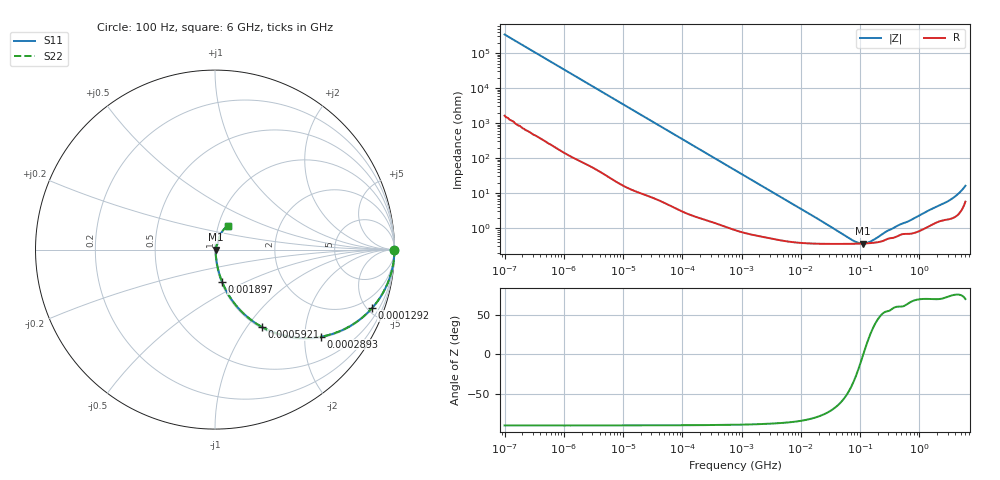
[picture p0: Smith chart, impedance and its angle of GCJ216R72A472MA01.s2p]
!Murata Part Number: GCJ216R72A472MA01
!These Parameters are Measured in Series Mode Connection
!Data Generated on Mar 13, 2026
!  o--ll--o
!Port1  Port2
!  o------o
!Operation Temp=25[degC], DC Bias Voltage=0[V]
!Freq. Start=100[Hz] Stop=6[GHz] 401[Steps]
# Hz S RI R 50
!Freq.(Hz) S11(Real) S11(Imag) S21(Real) S21(Imag) S12(Real) S12(Imag) S22(Real) S22(Imag)
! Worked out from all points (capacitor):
!   401 points, 100 Hz to 6 GHz, reference 50 ohm
!   read as one part in series: C = 4.69 nF near 109 Hz
!   lowest |Z| = 363 mohm at 111.6 MHz (marker M1)
!   series resonance near 113.6 MHz, so ESL is about 420 pH
!   S11 on the Smith chart (normalised r, x): 100 Hz: open; 129.2 kHz: 1.05, -5.37; 289.3 kHz: 1.03, -2.41; 592.1 kHz: 1.02, -1.18; 1.897 MHz: 1.01, -0.37; 6 GHz: 1.11, +0.30
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100  1 -0.000295  1.5e-06 0.000295  1.5e-06 0.000295  1 -0.000295
2008  0.9999 -0.00587  6.11e-05 0.00587  6.11e-05 0.00587  0.9999 -0.00587
12592  0.9985 -0.0366  0.00152 0.0366  0.00152 0.0366  0.9985 -0.0366
40335  0.9857 -0.1151  0.0143 0.1151  0.0143 0.1151  0.9857 -0.1151
78952  0.949 -0.216  0.051 0.216  0.051 0.216  0.949 -0.216
129199  0.8759 -0.3251  0.1241 0.3251  0.1241 0.3251  0.8759 -0.3251
193316  0.7612 -0.421  0.2388 0.421  0.2388 0.421  0.7612 -0.421
289253  0.5907 -0.4852  0.4093 0.4852  0.4093 0.4852  0.5907 -0.4852
413847  0.4172 -0.4856  0.5828 0.4856  0.5828 0.4856  0.4172 -0.4856
592111  0.2628 -0.4316  0.7372 0.4316  0.7372 0.4316  0.2628 -0.4316
774597  0.1751 -0.3705  0.8249 0.3705  0.8249 0.3705  0.1751 -0.3705
1159002  0.0899 -0.2744  0.9101 0.2744  0.9101 0.2744  0.0899 -0.2744
1896632  0.0389 -0.178  0.9611 0.178  0.9611 0.178  0.0389 -0.178
4643984  0.0102 -0.0756  0.9898 0.0756  0.9898 0.0756  0.0102 -0.0756
1.555665e7  0.00412 -0.0225  0.9959 0.0225  0.9959 0.0225  0.00412 -0.0225
7.455971e7  0.00355 -0.00273  0.9964 0.00273  0.9964 0.00273  0.00355 -0.00273
1.115611e8  0.00361 -0.000115  0.9964 0.000115  0.9964 0.000115  0.00361 -0.000115
1.526266e8  0.00373 0.0019  0.9963 -0.0019  0.9963 -0.0019  0.00373 0.0019
3.124326e8  0.00513 0.00714  0.9949 -0.00714  0.9949 -0.00714  0.00513 0.00714
2.931063e9  0.0199 0.0516  0.9801 -0.0516  0.9801 -0.0516  0.0199 0.0516
4.193612e9  0.0277 0.0782  0.9723 -0.0782  0.9723 -0.0782  0.0277 0.0782
6e9  0.0729 0.1331  0.9271 -0.1331  0.9271 -0.1331  0.0729 0.1331
